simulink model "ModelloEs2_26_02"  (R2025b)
settings: Solver=FixedStepAuto  StartTime=0.0  StopTime=Tsim  FixedStep=step  RelTol=1e-3
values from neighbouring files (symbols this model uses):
  a = 5    [ScriptEs2_26_02.m]    (also in ScriptEs2_27_02.m = 25)
  x0 = 1    [ScriptEs2_26_02.m]    (also in ScriptEs2_27_02.m = 2)
  y0 = -1    [ScriptEs2_26_02.m]    (also in ScriptEs2_27_02.m)
  ypunto0 = 0    [ScriptEs2_26_02.m]

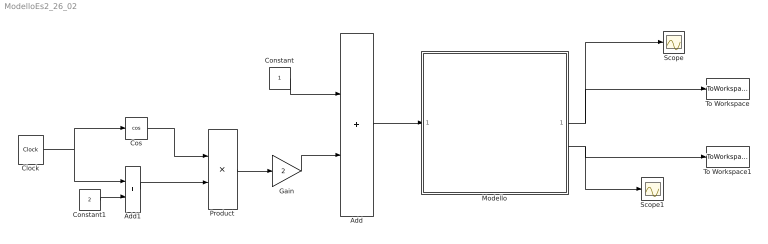
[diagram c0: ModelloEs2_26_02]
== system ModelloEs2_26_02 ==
  Add : Sum
  Add1 : Sum
  Clock : Clock
  Constant : Constant
  Constant1 : Constant  Value=2
  Cos : Trigonometry  Operator=cos
  Gain : Gain  Gain=2
  Modello : Subsystem
  Product : Product  Inputs=*/
  Scope : Scope
  Scope1 : Scope
  To Workspace : ToWorkspace  VariableName=x  SaveFormat=Timeseries  SampleTime=-1
  To Workspace1 : ToWorkspace  VariableName=y  SaveFormat=Timeseries  SampleTime=-1
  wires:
  Add/1 -> Modello/1(u(t))
  Constant/1 -> Add/1
  Gain/1 -> Add/2
  Product/1 -> Gain/1
  Cos/1 -> Product/1
  Clock/1 -> Add1/1, Cos/1
  Add1/1 -> Product/2
  Constant1/1 -> Add1/2
  Modello/1(x(t)) -> To Workspace/1, Scope/1
  Modello/2(y(t)) -> To Workspace1/1, Scope1/1

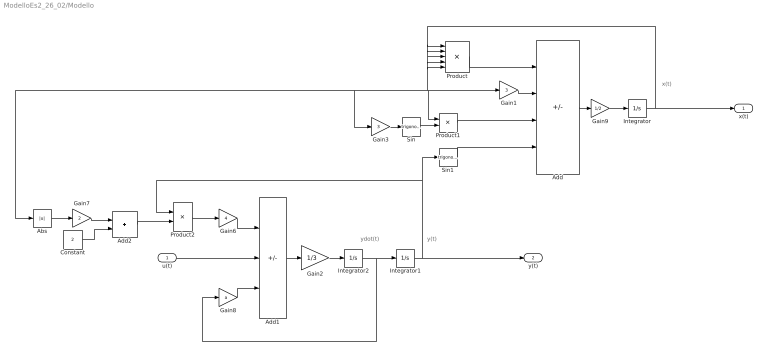
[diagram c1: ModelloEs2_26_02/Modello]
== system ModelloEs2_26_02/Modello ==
  note: y(t)
  note: ydot(t)
  note: x(t)
  u(t) : Inport
  Abs : Abs
  Add : Sum  Inputs=--+-
  Add1 : Sum  Inputs=-+-
  Add2 : Sum
  Constant : Constant  Value=2
  Gain1 : Gain  Gain=3
  Gain2 : Gain  Gain=1/3
  Gain3 : Gain  Gain=3
  Gain6 : Gain  Gain=4
  Gain7 : Gain  Gain=2
  Gain8 : Gain  Gain=a
  Gain9 : Gain  Gain=1/2
  Integrator : Integrator  InitialCondition=x0
  Integrator1 : Integrator  InitialCondition=y0
  Integrator2 : Integrator  InitialCondition=ypunto0
  Product : Product  Inputs=5
  Product1 : Product
  Product2 : Product  Inputs=*/
  Sin : Trigonometry
  Sin1 : Trigonometry
  x(t) : Outport  VectorParamsAs1DForOutWhenUnconnected=off
  y(t) : Outport  Port=2  VectorParamsAs1DForOutWhenUnconnected=off
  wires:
  Integrator/1 -> Product1/1, Gain1/1, Abs/1, Gain3/1, Product/5, Product/4, Product/3, Product/2, Product/1, x(t)/1
  Add/1 -> Gain9/1
  Product/1 -> Add/1
  Gain1/1 -> Add/2
  Product1/1 -> Add/3
  Sin/1 -> Product1/2
  Gain3/1 -> Sin/1
  Sin1/1 -> Add/4
  Integrator1/1 -> Product2/1, Sin1/1, y(t)/1
  Integrator2/1 -> Gain8/1, Integrator1/1
  Add1/1 -> Gain2/1
  u(t)/1 -> Add1/2
  Gain6/1 -> Add1/1
  Product2/1 -> Gain6/1
  Add2/1 -> Product2/2
  Constant/1 -> Add2/2
  Gain7/1 -> Add2/1
  Abs/1 -> Gain7/1
  Gain8/1 -> Add1/3
  Gain9/1 -> Integrator/1
  Gain2/1 -> Integrator2/1
